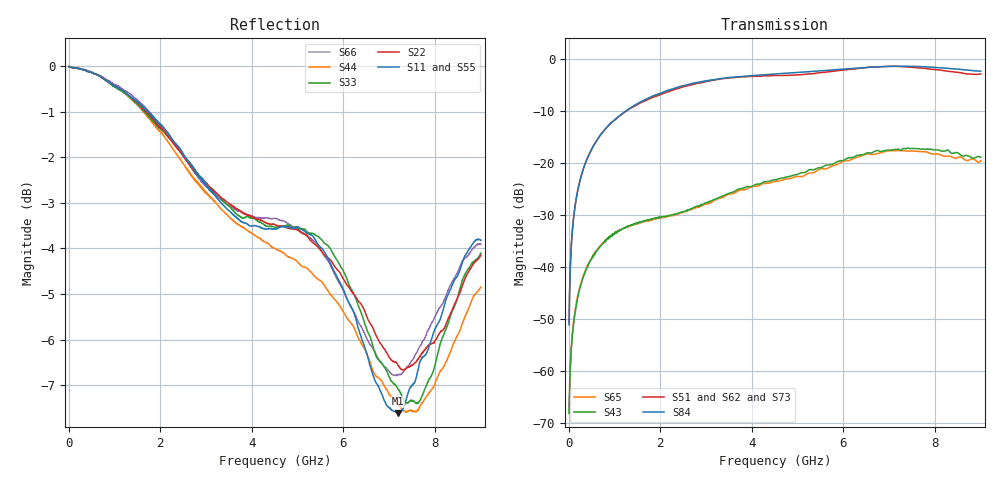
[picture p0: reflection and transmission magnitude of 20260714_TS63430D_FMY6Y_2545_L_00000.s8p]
# GHz S DB R 50
! CMT, SN0916, 25263762, 26.7.0
! Date: 15.07.2026 14:51:10
! Data: Format
! Freq S1.1:dB/Ang S1.2:dB/Ang S1.3:dB/Ang S1.4:dB/Ang S1.5:dB/Ang S1.6:dB/Ang S1.7:dB/Ang S1.8:dB/Ang
!  S2.1:dB/Ang S2.2:dB/Ang S2.3:dB/Ang S2.4:dB/Ang S2.5:dB/Ang S2.6:dB/Ang S2.7:dB/Ang S2.8:dB/Ang
!  S3.1:dB/Ang S3.2:dB/Ang S3.3:dB/Ang S3.4:dB/Ang S3.5:dB/Ang S3.6:dB/Ang S3.7:dB/Ang S3.8:dB/Ang
!  S4.1:dB/Ang S4.2:dB/Ang S4.3:dB/Ang S4.4:dB/Ang S4.5:dB/Ang S4.6:dB/Ang S4.7:dB/Ang S4.8:dB/Ang
!  S5.1:dB/Ang S5.2:dB/Ang S5.3:dB/Ang S5.4:dB/Ang S5.5:dB/Ang S5.6:dB/Ang S5.7:dB/Ang S5.8:dB/Ang
!  S6.1:dB/Ang S6.2:dB/Ang S6.3:dB/Ang S6.4:dB/Ang S6.5:dB/Ang S6.6:dB/Ang S6.7:dB/Ang S6.8:dB/Ang
!  S7.1:dB/Ang S7.2:dB/Ang S7.3:dB/Ang S7.4:dB/Ang S7.5:dB/Ang S7.6:dB/Ang S7.7:dB/Ang S7.8:dB/Ang
!  S8.1:dB/Ang S8.2:dB/Ang S8.3:dB/Ang S8.4:dB/Ang S8.5:dB/Ang S8.6:dB/Ang S8.7:dB/Ang S8.8:dB/Ang
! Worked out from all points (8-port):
!   2001 points, 10 MHz to 9 GHz, reference 50 ohm
!   strongest paths, dB at 10 MHz, 2.257 GHz, 4.505 GHz, 6.753 GHz, 9 GHz:
!     S84: -51.1, -5.7, -2.8, -1.4, -2.3
!     S51: -50.7, -6.0, -3.1, -1.5, -2.8
!     S62: -51.0, -5.9, -3.2, -1.8, -2.7
!     S73: -51.2, -6.0, -3.3, -1.7, -2.7
!     S43: -68.1, -29.9, -23.2, -17.6, -18.8
!     S65: -68.1, -30.1, -23.5, -18.1, -19.5
!   lowest |S11| = -7.6 dB at 7.184 GHz (marker M1), VSWR 2.43, Z = 21.5 - j9.33 ohm
!   |S11| at or under -10 dB: nowhere
